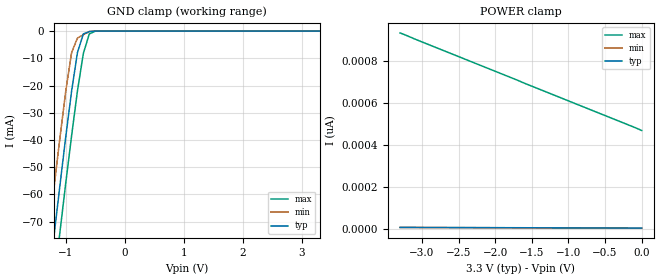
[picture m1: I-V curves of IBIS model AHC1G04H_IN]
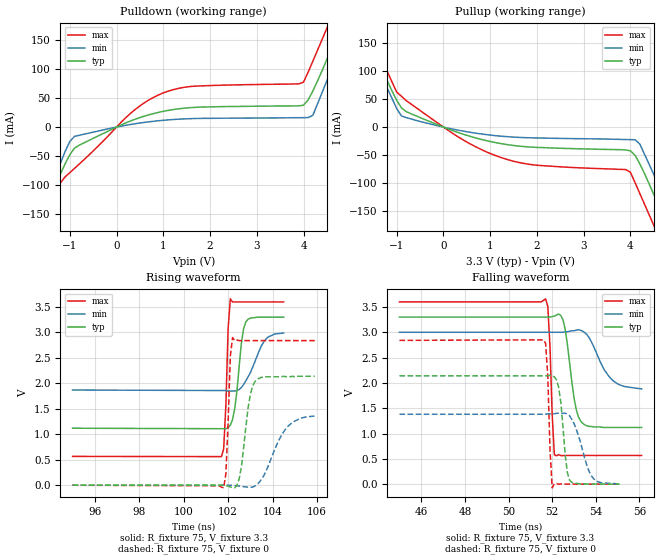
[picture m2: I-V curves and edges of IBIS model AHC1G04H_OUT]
| TEXAS INSTRUMENTS INCORPORATED
| Standard Linear and Logic Group
| IBIS Model of SN74AHC1G04H
| SINGLE INVERTER
| CMPAK-5 5-pin (DCK) Package
[IBIS Ver]   2.1
[Comment Char]  |_char
[File name]   ul04_3c.ibs
[File Rev]   2.0
[Date]   May 10, 2000
[Source]   Data created from SPICE simulations at Hitachi,Ltd.
[Notes]   The following is an IBIS List for the AHC1G04H.
|   Please contact sllibis@ti.com with questions and
|   comments concerning SLL IBIS models.
[Disclaimer] Property of Texas Instruments Incorporated.  Unauthorized
   reproduction and/or distribution is strictly prohibited.
   This product is protected under copyright law.
   Created 2000, (C) Copyright 2000, Texas Instruments Inc.,
   All Rights Reserved.
   UNLESS THERE IS A SIGNED, WRITTEN AGREEMENT TO THE
   CONTRARY, TEXAS INSTRUMENTS () IS PROVIDING THE IBIS
   MODELS  AND WITHOUT ANY WARRANTY, EXPRESSED OR
   IMPLIED.  TI assumes no liability for:
   1) the accuracy of the IBIS models provided to your
   company;
   2) the proper functioning of these IBIS Models in your
   design or for any resulting applications; or
   3) infringement of patents, copyrights or intellectual
   property rights resulting from your use of these IBIS
   models.
   TI provides IBIS Models as a service to our customers.
   You and your company shall not distribute, sell or give
   these models to anyone else without prior written
   permission from TI.
   TI reserves the right to make changes to our products or
   to discontinue any semiconductor product or service
   without notice, and advises our customers to obtain the
   latest version of relevant information to verify, before
   placing orders, that the information being relied on is
   current.
   Please be aware that your receipt and use of the IBIS
   information provided shall serve as acceptance of these
   terms and conditions.  If you do not accept these terms,
   you should return or destroy the IBIS models and any
   other accompanying information immediately.
|   Component AHC1G04H
[Component]   AHC1G04H
[Manufacturer]   Hitachi, Ltd.
[Package]
|   typ   min   max
R_pkg   0.090   0.051   0.105
L_pkg   1.500nH   0.940nH   1.700nH
C_pkg   0.170pF   0.110pF   0.360pF
[Pin]   signal_name   model_name   R_pin   L_pin   C_pin
1   NC   NC   0.098   1.590nH   0.110pF
2   A   AHC1G04H_IN   0.051   0.940nH   0.170pF
3   GND   GND   0.092   1.590nH   0.360pF
4   Y   AHC1G04H_OUT   0.105   1.700nH   0.110pF
5   VCC   POWER   0.104   1.690nH   0.110pF
| Models and submodels in the file (2): AHC1G04H_IN (Input), AHC1G04H_OUT (Output)
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|   Model AHC1G04H_IN
[Model]   AHC1G04H_IN
Model_type  Input
Polarity   Inverting
Vinl = 0.99
Vinh = 2.31
| variable   typ   min   max
C_comp   1.80pF   1.73pF   1.97pF
[Temperature Range]   25   85   -40
[Voltage Range]   3.3   3.0   3.6
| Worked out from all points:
|   GND clamp passes 1 mA (typ) near -0.70 V on its own axis
[GND Clamp]
|   Voltage   I(typ)   I(min)   I(max)
-3.3V     -486mA     -469mA     -503mA
-1.3V     -94.6mA    -76.9mA    -112mA
-1.2V     -75.8mA    -58.1mA    -93.1mA
-1.1V     -57.3mA    -39.8mA    -74.5mA
-1V       -39.2mA    -22.4mA    -56.2mA
-900mV    -22.2mA    -7.98mA    -38.6mA
-800mV    -7.87mA    -2.53mA    -22mA
-700mV    -1.03mA    -1.34mA    -8.2mA
-600mV    -206uA     -154uA     -1.06mA
-500mV    -11.2uA    -2.6uA     -57.2uA
3.3V      3.55pA     3.3pA      469pA
[POWER Clamp]
|   Voltage   I(typ)   I(min)   I(max)
-3.3V     7pA        6.6pA      934pA
-1.6V     5.23pA     4.9pA      694pA
-100mV    3.66pA     3.4pA      484pA
0V        3.55pA     3.3pA      469pA
|   Model AHC1G04H_OUT
[Model]   AHC1G04H_OUT
Model_type  Output
Polarity   Non-Inverting
Vmeas = 1.65
Cref = 15pf
| variable   typ   min   max
C_comp   3.84pF   3.72pF   3.96pF
[Temperature Range]   25   85   -40
[Voltage Range]   3.3   3.0   3.6
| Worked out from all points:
|   slope of the pulldown table from 0 to 0.495 V, typ, clamps not added: 30.4 ohm
|   slope of the pullup table from 0 to 0.495 V, typ, clamps not added: 34 ohm
|   rising waveform, R_fixture 75, V_fixture 3.3: 20-80 % time 310ps typ, 682ps min, 141ps max; typ from 1.12 V to 3.3 V
|   falling waveform, R_fixture 75, V_fixture 3.3: 20-80 % time 405ps typ, 814ps min, 160ps max; typ from 3.3 V to 1.12 V
|   falling waveform, R_fixture 75, V_fixture 0: 20-80 % time 275ps typ, 582ps min, 139ps max; typ from 2.14 V to 0 V
|   rising waveform, R_fixture 75, V_fixture 0: 20-80 % time 357ps typ, 860ps min, 146ps max; typ from 0 V to 2.14 V
[Pulldown]
|   Voltage   I(typ)   I(min)   I(max)
-3.3V     -489mA     -473mA     -506mA
-1.8V     -194mA     -179mA     -211mA
-1.6V     -156mA     -142mA     -173mA
-1.2V     -81mA      -62.6mA    -96.6mA
-900mV    -36.6mA    -16.1mA    -71.6mA
1V        27.2mA     11.7mA     59.1mA
3.9V      36.7mA     16.2mA     74.7mA
4.1V      47mA       16.4mA     95.1mA
4.5V      117mA      80.2mA     171mA
4.8V      174mA      137mA      229mA
5V        213mA      175mA      268mA
6.6V      528mA      491mA      584mA
[Pullup]
|   Voltage   I(typ)   I(min)   I(max)
-3.3V     491mA      474mA      508mA
-1.8V     196mA      179mA      214mA
-1.6V     157mA      141mA      175mA
-1V       47.9mA     33.1mA     62.4mA
-900mV    34.5mA     20mA       55.1mA
1.2V      -29mA      -16mA      -53.4mA
3.9V      -40.8mA    -22.2mA    -75.7mA
4.2V      -65.2mA    -30mA      -118mA
4.5V      -120mA     -84.4mA    -175mA
4.8V      -177mA     -138mA     -233mA
5V        -216mA     -177mA     -272mA
6.6V      -533mA     -494mA     -589mA
[Ramp]
| variable   typ   min   max
dV/dt_r   1.28E+00/3.50E-10   8.28E-01/8.80E-10   1.71E+00/1.40E-10
dV/dt_f   1.31E+00/4.00E-10   6.76E-01/8.20E-10   1.82E+00/1.50E-10
R_load = 75
[Rising Waveform]
R_fixture = 75
V_fixture = 3.3
V_fixture_min = 3.0
V_fixture_max = 3.6
|   Time   V(typ)   V(min)   V(max)
95ns      1.12V      1.87V      566mV
101.7ns   1.11V      1.86V      562mV
101.8ns   1.11V      1.86V      710mV
101.9ns   1.11V      1.86V      1.57V
102ns     1.13V      1.85V      3.07V
102.1ns   1.18V      1.85V      3.66V
102.3ns   1.51V      1.85V      3.6V
102.8ns   3.21V      2.05V      3.6V
103.7ns   3.3V       2.87V      3.6V
104.5ns   3.3V       2.99V      3.6V
[Falling Waveform]
R_fixture = 75
V_fixture = 3.3
V_fixture_min = 3.0
V_fixture_max = 3.6
|   Time   V(typ)   V(min)   V(max)
45ns      3.3V       3V         3.6V
51.7ns    3.3V       3V         3.66V
51.8ns    3.3V       3V         3.51V
52ns      3.31V      3V         1.37V
52.1ns    3.32V      3V         582mV
52.5ns    3.24V      3V         564mV
53ns      1.71V      3.03V      566mV
53.3ns    1.25V      3.04V      566mV
54.7ns    1.12V      2.08V      566mV
56.1ns    1.12V      1.88V      566mV
[Falling Waveform]
R_fixture = 75
V_fixture = 0
|   Time   V(typ)   V(min)   V(max)
45ns      2.14V      1.38V      2.84V
51.6ns    2.14V      1.38V      2.85V
51.7ns    2.14V      1.38V      2.78V
51.8ns    2.14V      1.39V      2.12V
51.9ns    2.15V      1.39V      689mV
52ns      2.14V      1.39V      -73.7mV
52.3ns    1.91V      1.4V       -2.97mV
52.8ns    76.5mV     1.35V      137uV
53.8ns    872uV      163mV      70uV
55.1ns    -59uV      3.66mV     -37uV
[Rising Waveform]
R_fixture = 75
V_fixture = 0
|   Time   V(typ)   V(min)   V(max)
95ns      0V         0V         0V
101.8ns   -2.69mV    1.41mV     -51.5mV
101.9ns   -8.6mV     1.7mV      223mV
102.1ns   -34.6mV    -111uV     2.53V
102.2ns   -49.3mV    -2.37mV    2.9V
102.5ns   129mV      -15.8mV    2.84V
102.9ns   1.52V      -38mV      2.84V
103.2ns   2.03V      -17.9mV    2.84V
104.6ns   2.13V      1.11V      2.84V
105.9ns   2.14V      1.36V      2.84V
